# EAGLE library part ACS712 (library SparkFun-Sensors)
ACS712 Hall-effect-based isolated linear current sensor Datasheet SparkFun Products SparkFun Low Current Sensor Breakout - ACS712 (SEN-08883)
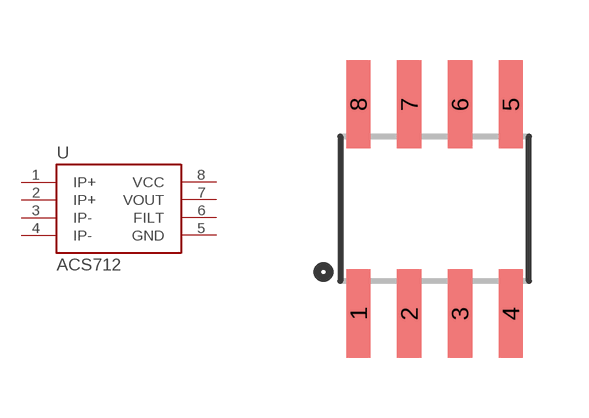
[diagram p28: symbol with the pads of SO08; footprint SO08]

Designator prefix -

## ACS712 (PROD_ID: IC-08964; VALUE: ACS712)  [SO08]
1  IP+
2  IP+
3  IP-
4  IP-
5  GND
6  FILT
7  VOUT
8  VCC

## Footprint SO08 (pad centres in mm)
Small Outline Package Fits JEDEC packages (narrow SOIC-8)
smd 0.61 x 2.21: 1 -1.905,-2.616; 2 -0.635,-2.616; 3 0.635,-2.616; 4 1.905,-2.616; 5 1.905,2.616; 6 0.635,2.616; 7 -0.635,2.616; 8 -1.905,2.616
